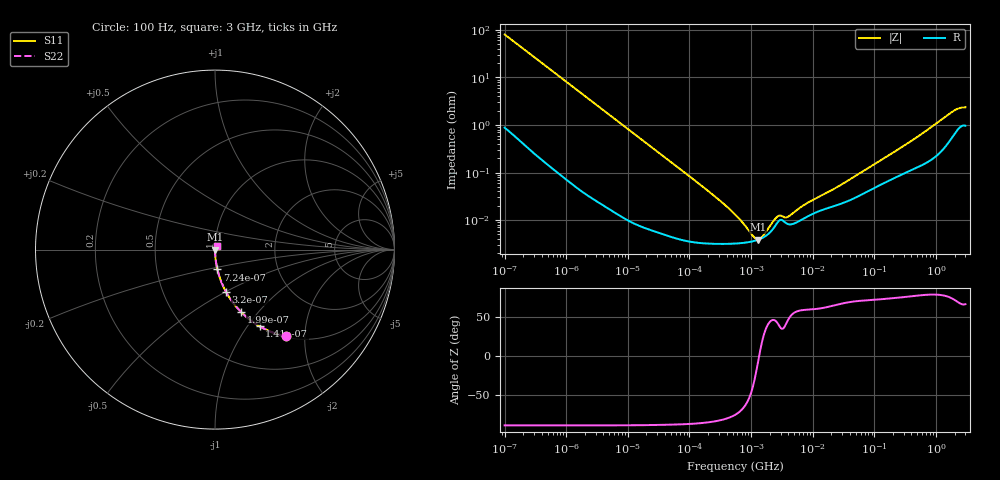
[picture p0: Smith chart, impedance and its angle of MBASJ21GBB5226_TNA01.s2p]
! MBASJ21GBB5226_TNA01  S-PARAMETER MODEL  ( Standard Model )
! Model Generated by TAIYO YUDEN Corporation (http://www.ty-top.com)
! Version 2.0
! TAIYO YUDEN Control No. 230609
! Copyright(c) 2012 TAIYO YUDEN CO.,LTD. All Rights Reserved.
! Product Description (link to TY-COMPAS)
! https://ds.yuden.co.jp/TYCOMPAS/or/detail?pn=MBASJ21GBB5226MTNA01&u=M
! Products Name : Multilayer Ceramic Capacitors
! Characteristics :
!  Capacitance : 22 [uF] , Rated Voltage : 6.3 [V] , TCC : X5R
!  Case Size : 2.0 x 1.25 / 0.079 x 0.049 [mm/inch] , Thickness : 1.25 / 0.049 [mm/inch]
!  (Conditions: Temperature = 25 [degC] , DC Bias Voltage = 0 [V])
! External Node Assignments :
!  1  o---| |---o  2
! GND o---------o GND
! Frequency Range : 100Hz  -  3GHz  [ 401 STEP ]
# MHZ S RI R 50
! Freq[MHz].  S11 Real  S11 Imag  S21 Real  S21 Imag  S12 Real  S12 Imag  S22 Real  S22 Imag
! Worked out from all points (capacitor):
!   401 points, 100 Hz to 3 GHz, reference 50 ohm
!   read as one part in series: C = 19.8 uF near 109 Hz
!   lowest |Z| = 3.89 mohm at 1.295 MHz (marker M1)
!   series resonance near 1.353 MHz, so ESL is about 700 pH
!   S11 on the Smith chart (normalised r, x): 100 Hz: 1.02, -1.61; 141 Hz: 1.01, -1.14; 199 Hz: 1.01, -0.81; 320 Hz: 1.00, -0.51; 724 Hz: 1.00, -0.22; 3 GHz: 1.02, +0.04
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0.0001  0.3934 -0.4831  0.6066 0.4831  0.6066 0.4831  0.3934 -0.4831
0.000141  0.2481 -0.4267  0.7519 0.4267  0.7519 0.4267  0.2481 -0.4267
0.000199  0.1437 -0.3459  0.8563 0.3459  0.8563 0.3459  0.1437 -0.3459
0.00032  0.0622 -0.237  0.9378 0.237  0.9378 0.237  0.0622 -0.237
0.000724  0.0134 -0.1107  0.9866 0.1107  0.9866 0.1107  0.0134 -0.1107
0.001788  0.00248 -0.0456  0.9975 0.0456  0.9975 0.0456  0.00248 -0.0456
0.031977  6.03e-05 -0.00259  0.9999 0.00259  0.9999 0.00259  6.03e-05 -0.00259
0.221826  3.19e-05 -0.000367  1 0.000367  1 0.000367  3.19e-05 -0.000367
0.547723  3.2e-05 -0.000128  1 0.000128  1 0.000128  3.2e-05 -0.000128
0.623217  3.23e-05 -0.000106  1 0.000106  1 0.000106  3.23e-05 -0.000106
0.709116  3.28e-05 -8.59e-05  1 8.59e-05  1 8.59e-05  3.28e-05 -8.59e-05
1.295438  3.85e-05 -5.48e-06  1 5.48e-06  1 5.48e-06  3.85e-05 -5.48e-06
2.171352  6.05e-05 6.11e-05  0.9999 -6.11e-05  0.9999 -6.11e-05  6.05e-05 6.11e-05
2.93481  9.98e-05 7.46e-05  0.9999 -7.46e-05  0.9999 -7.46e-05  9.98e-05 7.46e-05
3.79959  8.41e-05 7.74e-05  0.9999 -7.74e-05  0.9999 -7.74e-05  8.41e-05 7.74e-05
9.794414  0.000133 0.000224  0.9999 -0.000224  0.9999 -0.000224  0.000133 0.000224
27.51729  0.000216 0.000486  0.9998 -0.000486  0.9998 -0.000486  0.000216 0.000486
175.1444  0.000684 0.00224  0.9993 -0.00224  0.9993 -0.00224  0.000684 0.00224
536.3016  0.00137 0.00583  0.9986 -0.00583  0.9986 -0.00583  0.00137 0.00583
1868.531  0.006 0.0182  0.994 -0.0182  0.994 -0.0182  0.006 0.0182
2317.205  0.00866 0.0203  0.9913 -0.0203  0.9913 -0.0203  0.00866 0.0203
3000  0.01 0.0211  0.99 -0.0211  0.99 -0.0211  0.01 0.0211
